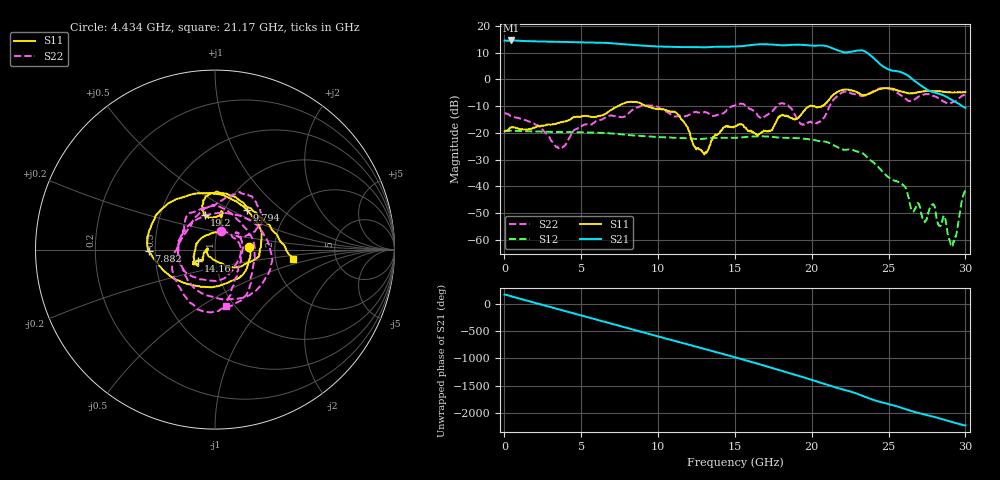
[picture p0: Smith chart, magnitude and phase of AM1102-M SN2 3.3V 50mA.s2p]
!Agilent Technologies,E8364B,MY43040894,A.07.50.67
!Agilent E8364B: A.07.50.67
!Date: Monday, May 24, 2021 14:26:21
!Correction: S11(Full 2 Port(1,2))
!S21(Full 2 Port(1,2))
!S12(Full 2 Port(1,2))
!S22(Full 2 Port(1,2))
!S2P File: Measurements: S11, S21, S12, S22:
# Hz S  dB  R 50
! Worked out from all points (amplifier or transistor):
!   1601 points, 10 MHz to 30 GHz, reference 50 ohm
!   highest |S21| = 14.6 dB at 422.4 MHz (marker M1)
!   |S21| within 3 dB of that: start of sweep to 21.37 GHz
!   unconditionally stable (mu >= 1): start of sweep to end of sweep
!   at 4.996 GHz: K = 1.20, MAG = 14.1 dB, |S12| = -19.8 dB
!   at 15.01 GHz: K = 1.46, MAG = 13.1 dB, |S12| = -21.9 dB
!   at 30 GHz: K = 102.09, MAG = -7.6 dB, |S12| = -41.7 dB
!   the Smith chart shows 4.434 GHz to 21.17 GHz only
!   S11 on the Smith chart (normalised r, x): 4.434 GHz: 1.47, +0.05; 7.882 GHz: 0.46, -0.01; 9.794 GHz: 1.27, +0.61; 14.16 GHz: 0.82, -0.10; 19.2 GHz: 0.83, +0.34; 21.17 GHz: 2.50, -0.33
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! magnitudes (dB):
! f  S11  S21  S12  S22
! 10 MHz  -19.5  14.5  -19.1  -12.6
! 422.4 MHz  -17.9  14.6  -19.2  -13.7
! 3.515 GHz  -16.3  14.1  -19.7  -25.8
! 4.434 GHz  -14.3  14.0  -19.8  -19.4
! 5.015 GHz  -13.8  13.9  -19.8  -17.5
! 7.882 GHz  -8.7  13.1  -20.7  -13.7
! 9.794 GHz  -11.0  12.4  -21.5  -9.9
! 10.02 GHz  -11.1  12.3  -21.6  -10.4
! 11.24 GHz  -12.8  12.1  -21.9  -13.8
! 13.02 GHz  -28.1  12.0  -22.2  -12.2
! 14.16 GHz  -18.9  12.3  -21.9  -12.9
! 15.01 GHz  -17.6  12.3  -21.9  -9.8
! 16.75 GHz  -19.7  13.2  -21.3  -14.5
! 18.21 GHz  -13.5  12.8  -21.9  -9.1
! 19.2 GHz  -13.8  13.0  -22.0  -16.1
! 20.01 GHz  -10.0  12.6  -22.6  -16.2
! 21.17 GHz  -7.2  12.0  -23.9  -9.9
! 25.01 GHz  -3.3  3.7  -36.7  -3.5
! 27.32 GHz  -4.5  -3.1  -53.0  -5.6
! 27.9 GHz  -4.4  -4.8  -46.7  -6.2
! 29.12 GHz  -5.0  -7.7  -62.2  -8.7
! 30 GHz  -4.7  -10.6  -41.7  -6.0
